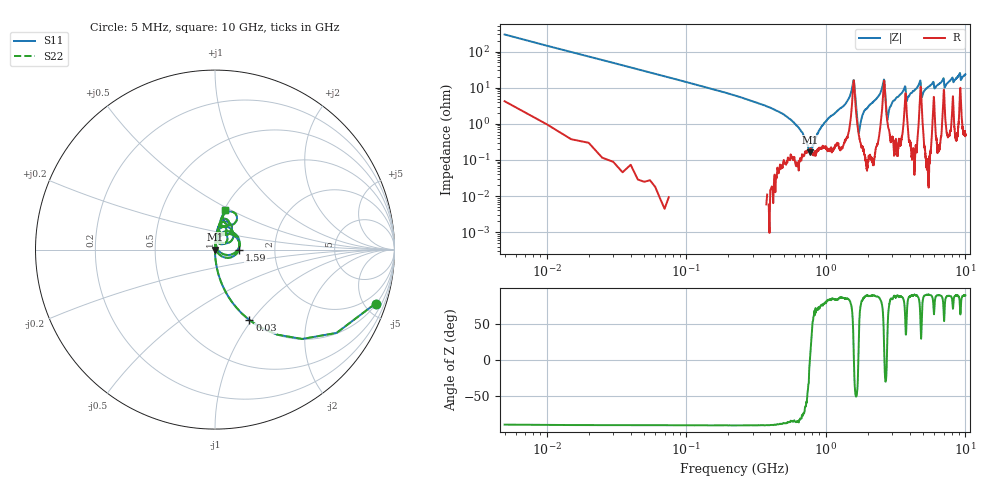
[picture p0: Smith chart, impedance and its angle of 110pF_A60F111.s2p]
! Amotech Co.,Ltd.
! http://www.amotech.co.kr/
! Part Number: A60F111
! These Parameters are Measured in Series Mode Connection
! Operation Temp=25[degC], DC Bias Voltage=0[V]
! Freq. Start=5[MHz] Stop=10[GHz], 2000[Steps]
! Date: Monday, July 20, 2020, 03:45:02
# GHZ S RI R 50.000000
!Freq.(Hz) S11(Real) S11(Imag) S21(Real) S21(Imag) S12(Real) S12(Imag) S22(Real) S22(Imag)
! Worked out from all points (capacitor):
!   2000 points, 5 MHz to 10 GHz, reference 50 ohm
!   read as one part in series: C = 109 pF near 55 MHz
!   lowest |Z| = 162 mohm at 775 MHz (marker M1)
!   series resonance near 769.6 MHz, so ESL is about 390 pH
!   S11 on the Smith chart (normalised r, x): 5 MHz: 1.08, -5.93; 30 MHz: 1.00, -0.97; 1.59 GHz: 1.31, -0.01; 10 GHz: 1.01, +0.47
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0.005  0.8944 -0.3004  0.1056 0.3004  0.1056 0.3004  0.8944 -0.3004
0.03  0.1914 -0.3925  0.8086 0.3925  0.8086 0.3925  0.1914 -0.3925
0.11  0.0162 -0.1278  0.9838 0.1278  0.9838 0.1278  0.0162 -0.1278
0.575  0.00137 -0.0118  0.9986 0.0118  0.9986 0.0118  0.00137 -0.0118
0.775  0.00159 0.000268  0.9984 -0.000268  0.9984 -0.000268  0.00159 0.000268
1  0.00249 0.0112  0.9975 -0.0112  0.9975 -0.0112  0.00249 0.0112
1.59  0.1329 -0.00342  0.8671 0.00342  0.8671 0.00342  0.1329 -0.00342
1.675  0.0114 -0.0111  0.9886 0.0111  0.9886 0.0111  0.0114 -0.0111
1.74  0.00385 0.00565  0.9961 -0.00565  0.9961 -0.00565  0.00385 0.00565
1.895  0.00191 0.0232  0.9981 -0.0232  0.9981 -0.0232  0.00191 0.0232
2.59  0.1016 0.0946  0.8984 -0.0946  0.8984 -0.0946  0.1016 0.0946
2.765  0.0103 0.00741  0.9897 -0.00741  0.9897 -0.00741  0.0103 0.00741
3.005  0.00569 0.0394  0.9943 -0.0394  0.9943 -0.0394  0.00569 0.0394
3.34  0.00731 0.0585  0.9927 -0.0585  0.9927 -0.0585  0.00731 0.0585
3.68  0.0446 0.0914  0.9554 -0.0914  0.9554 -0.0914  0.0446 0.0914
3.815  0.0175 0.0395  0.9825 -0.0395  0.9825 -0.0395  0.0175 0.0395
4.725  0.0649 0.1274  0.9351 -0.1274  0.9351 -0.1274  0.0649 0.1274
4.875  0.0272 0.0443  0.9728 -0.0443  0.9728 -0.0443  0.0272 0.0443
5.005  0.0106 0.0732  0.9894 -0.0732  0.9894 -0.0732  0.0106 0.0732
6.67  0.0229 0.135  0.9771 -0.135  0.9771 -0.135  0.0229 0.135
8.335  0.0322 0.1523  0.9678 -0.1523  0.9678 -0.1523  0.0322 0.1523
10  0.0559 0.2191  0.9441 -0.2191  0.9441 -0.2191  0.0559 0.2191
